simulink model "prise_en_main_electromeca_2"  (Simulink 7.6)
settings: Solver=ode15s  StartTime=0.0  StopTime=60  RelTol=1e-3
InitFcn:
  | U0=12;       % échelon d'entrée en V
StopFcn:
  | close all
  | % lecture du fichier binaire
  | load DC_Motor.mat
  | 
  | % trace de la tension et du courant d’induit
  | plotyy(x(1,:),x(2,:),x(1,:),x(3,:))
  | title('Tension et courant d''induit')
  | grid
  | gtext('Tension d''induit en V')
  | gtext('Courant d''induit en A')
  | 
  | figure
  | plotyy(x(1,:),x(4,:),x(1,:),x(5,:))
  | title('Vitesse en rad/s et position angulaire en rad')
  | grid
  | gtext('position angulaire')
  | gtext('vitesse angulaire')
libraries: fl_lib x12, nesl_utility x6, elec_lib x1

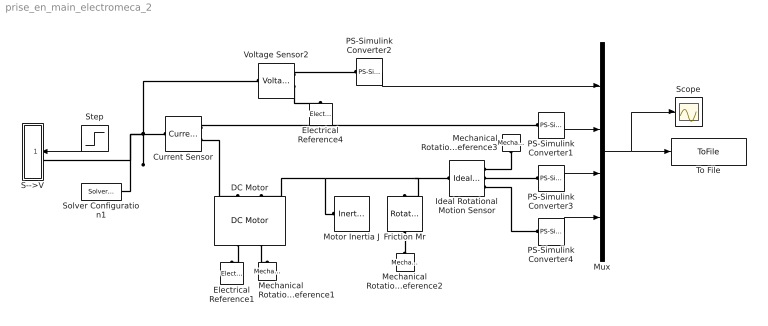
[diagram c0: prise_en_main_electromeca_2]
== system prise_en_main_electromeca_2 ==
  Current Sensor : fl_lib/Electrical/Electrical Sensors/Current Sensor  DialogController=NetworkEngine.DynNeDlgSource  SystemSampleTime=-1  i1_Log=off  v1_Log=off  LocalVarNames=|i1|v1  LocalVarDescs=|i1|v1  LocalVarLogging=[0 0]
  DC Motor : elec_lib/Actuators & Drivers/Rotational Actuators/DC Motor  DialogController=NetworkEngine.DynNeDlgSource  SystemSampleTime=-1  parameterization=1  Ra=3.9 Ohm  La=1.2e-05 H  emf_or_torque=1  Kv=7.2e-05 V/rpm  Ki=6.876e-04 N*m/A  T_stall=2.4e-04 N*m  w_max=1.91e+04 rpm  w_rated=1.5e+04 rpm  P_rated=0.08 W  V_rated=1.5 V  J=0.01 g*cm^2  lam=1e-08 N*m/(rad/s)  speed0=0 rpm  current_Log=off  voltage_Log=off  power_Log=off  i2r_Log=off  torque_Log=off  speed_Log=off  LocalVarNames=|current|voltage|power|i2r|torque|speed  LocalVarDescs=|Current (A)|Voltage (V)|Power (W)|Electrical losses (W)|Torque (Nm)|Angular speed (rad/s)  LocalVarLogging=[0 0 0 0 0 0]
  Electrical Reference1 : fl_lib/Electrical/Electrical Elements/Electrical Reference  DialogController=NetworkEngine.DynNeDlgSource  SystemSampleTime=-1  i_Log=off  LocalVarNames=|i  LocalVarDescs=|i  LocalVarLogging=[]
  Electrical Reference4 : fl_lib/Electrical/Electrical Elements/Electrical Reference  DialogController=NetworkEngine.DynNeDlgSource  SystemSampleTime=-1  i_Log=off  LocalVarNames=|i  LocalVarDescs=|i  LocalVarLogging=[]
  Friction Mr : fl_lib/Mechanical/Rotational Elements/Rotational Friction  DialogController=NetworkEngine.DynNeDlgSource  SystemSampleTime=-1  brkwy_trq=0.02e-3 N*m  Col_trq=0.02e-3 N*m  visc_coef=0 N*m/(rad/s)  trans_coef=10 s/rad  vel_thr=0.1 rad/s  t_Log=off  w_Log=off  LocalVarNames=|friction_torque|rel_velocity|power  LocalVarDescs=|Friction torque (N*m)|Relative velocity (rad/s)|Power (W)  LocalVarLogging=[0 0 0]
  Ideal Rotational Motion Sensor : fl_lib/Mechanical/Mechanical Sensors/Ideal Rotational Motion Sensor  DialogController=NetworkEngine.DynNeDlgSource  SystemSampleTime=-1  offset=0 rad  w_Log=off  t_Log=off  phi_Log=off  LocalVarNames=|w|t|phi  LocalVarDescs=|w|t|phi  LocalVarLogging=[0 0 0]
  Mechanical Rotational Reference1 : fl_lib/Mechanical/Rotational Elements/Mechanical Rotational Reference  DialogController=NetworkEngine.DynNeDlgSource  SystemSampleTime=-1  t_Log=off  LocalVarNames=|t  LocalVarDescs=|t  LocalVarLogging=0
  Mechanical Rotational Reference2 : fl_lib/Mechanical/Rotational Elements/Mechanical Rotational Reference  DialogController=NetworkEngine.DynNeDlgSource  SystemSampleTime=-1  t_Log=off  LocalVarNames=|t  LocalVarDescs=|t  LocalVarLogging=0
  Mechanical Rotational Reference3 : fl_lib/Mechanical/Rotational Elements/Mechanical Rotational Reference  DialogController=NetworkEngine.DynNeDlgSource  SystemSampleTime=-1  t_Log=off  LocalVarNames=|t  LocalVarDescs=|t  LocalVarLogging=0
  Motor Inertia J : fl_lib/Mechanical/Rotational Elements/Inertia  DialogController=NetworkEngine.DynNeDlgSource  SystemSampleTime=-1  inertia=10 g*cm^2  initial_velocity=0 rad/s  t_Log=off  LocalVarNames=|torque|velocity  LocalVarDescs=|Inertia torque (N*m)|Inertia absolute velocity (rad/s)  LocalVarLogging=[0 0]
  Mux : Mux
  PS-Simulink Converter1 : nesl_utility/PS-Simulink Converter  DialogController=NetworkEngine.DynNeUtilDlgSource  SystemSampleTime=-1  PhysicalDomain=network_engine_domain  LeftPortType=input  RightPortType=output  SubClassName=ps_output  Unit=A  AffineConversion=off
  PS-Simulink Converter2 : nesl_utility/PS-Simulink Converter  DialogController=NetworkEngine.DynNeUtilDlgSource  SystemSampleTime=-1  PhysicalDomain=network_engine_domain  LeftPortType=input  RightPortType=output  SubClassName=ps_output  Unit=1  AffineConversion=off
  PS-Simulink Converter3 : nesl_utility/PS-Simulink Converter  DialogController=NetworkEngine.DynNeUtilDlgSource  SystemSampleTime=-1  PhysicalDomain=network_engine_domain  LeftPortType=input  RightPortType=output  SubClassName=ps_output  Unit=rad/s  AffineConversion=off
  PS-Simulink Converter4 : nesl_utility/PS-Simulink Converter  DialogController=NetworkEngine.DynNeUtilDlgSource  SystemSampleTime=-1  PhysicalDomain=network_engine_domain  LeftPortType=input  RightPortType=output  SubClassName=ps_output  Unit=rad  AffineConversion=off
  S-->V : Subsystem
  Scope : Scope
  Solver Configuration1 : nesl_utility/Solver Configuration  DialogController=NetworkEngine.DynNeUtilDlgSource  SystemSampleTime=-1  PhysicalDomain=network_engine_domain  LeftPortType=input  RightPortType=generic  SubClassName=solver  Accelerate=off  Profile=off  ResidualTolerance=1e-9  MaxNonlinIter=12  MaxModeIter=2  DoFixedCost=off  UseLocalSampling=off  DoDC=off  LinearAlgebra=Sparse  LocalSolverSampleTime=.001  LocalSolverChoice=NE_BACKWARD_EULER_ADVANCER  UseLocalSolver=off
  Step : Step  Time=2  After=U0  SampleTime=0
  To File : ToFile  Filename=DC_Motor.mat  MatrixName=x
  Voltage Sensor2 : fl_lib/Electrical/Electrical Sensors/Voltage Sensor  DialogController=NetworkEngine.DynNeDlgSource  SystemSampleTime=-1  i1_Log=off  v1_Log=off  LocalVarNames=|i1|v1  LocalVarDescs=|i1|v1  LocalVarLogging=[]
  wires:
  PS-Simulink Converter2/1 -> Mux/1
  Step/1 -> S-->V/1(S)
  PS-Simulink Converter1/1 -> Mux/2
  Mux/1 -> Scope/1, To File/1
  PS-Simulink Converter3/1 -> Mux/3
  PS-Simulink Converter4/1 -> Mux/4
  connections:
  Voltage Sensor2/RConn1 -- PS-Simulink Converter2/LConn1
  S-->V/LConn1 -- Solver Configuration1/RConn1 -- Voltage Sensor2/LConn1 -- Current Sensor/LConn1
  Voltage Sensor2/RConn2 -- Electrical Reference4/LConn1
  DC Motor/RConn1 -- Electrical Reference1/LConn1
  Current Sensor/RConn1 -- PS-Simulink Converter1/LConn1
  Current Sensor/RConn2 -- DC Motor/LConn1
  DC Motor/RConn2 -- Mechanical Rotational Reference1/LConn1
  Mechanical Rotational Reference3/LConn1 -- Ideal Rotational Motion Sensor/RConn1
  Ideal Rotational Motion Sensor/LConn1 -- DC Motor/LConn2 -- Motor Inertia J/LConn1 -- Friction Mr/LConn1
  Ideal Rotational Motion Sensor/RConn2 -- PS-Simulink Converter3/LConn1
  Ideal Rotational Motion Sensor/RConn3 -- PS-Simulink Converter4/LConn1
  Friction Mr/RConn1 -- Mechanical Rotational Reference2/LConn1

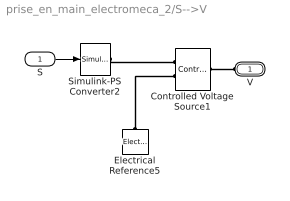
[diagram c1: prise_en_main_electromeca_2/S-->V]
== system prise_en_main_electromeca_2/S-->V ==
  S : Inport
  Controlled Voltage Source1 : fl_lib/Electrical/Electrical Sources/Controlled Voltage Source  DialogController=NetworkEngine.DynNeDlgSource  SystemSampleTime=-1  i_Log=off  v_Log=off  LocalVarNames=|current|voltage|power  LocalVarDescs=|Current (A)|Voltage (V)|Power (W)  LocalVarLogging=[0 0 0]
  Electrical Reference5 : fl_lib/Electrical/Electrical Elements/Electrical Reference  DialogController=NetworkEngine.DynNeDlgSource  SystemSampleTime=-1  i_Log=off  LocalVarNames=|i  LocalVarDescs=|i  LocalVarLogging=[]
  Simulink-PS Converter2 : nesl_utility/Simulink-PS Converter  DialogController=NetworkEngine.DynNeUtilDlgSource  SystemSampleTime=-1  PhysicalDomain=network_engine_domain  LeftPortType=input  RightPortType=output  SubClassName=ps_input  Unit=1  AffineConversion=off  InputFilterTimeConstant=.001  UdotUserProvided=0
  V : PMIOPort  Port=1  Side=Left
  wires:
  S/1 -> Simulink-PS Converter2/1
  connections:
  Simulink-PS Converter2/RConn1 -- Controlled Voltage Source1/RConn1
  Electrical Reference5/LConn1 -- Controlled Voltage Source1/RConn2
  V/RConn1 -- Controlled Voltage Source1/LConn1
